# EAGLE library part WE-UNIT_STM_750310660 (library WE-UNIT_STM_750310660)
Off-Line Transformer WE-Unit STM - Nominal input voltage: 85-265 VAC - Operating temperature: -40°C to +125 °C - Isolation voltage 4 kVAC -- Especially designed for several ICs from STMicroelectronics VIPer 17H -- Universal input -- Offline-switch mode power supplies
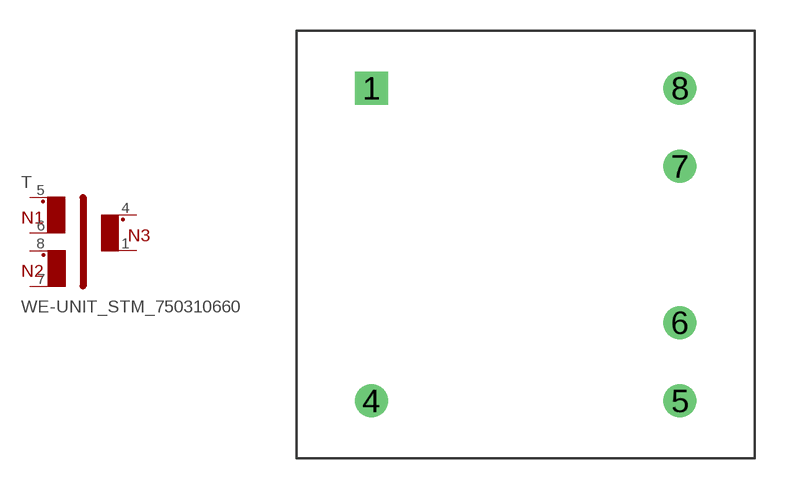
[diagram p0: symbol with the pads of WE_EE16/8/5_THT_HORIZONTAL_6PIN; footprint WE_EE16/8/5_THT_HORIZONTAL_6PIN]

Designator prefix T

## WE-UNIT_STM_750310660 (MPN: 750310660; OC_FARNELL: 1849043; OC_NEWARK: 13T9827; PACKAGE: EE16/8/5; SUPPLIER: Würth Elektronik eiSos GmbH)  [WE_EE16/8/5_THT_HORIZONTAL_6PIN]
1  5  pas
4  6  pas
5  1  pas
6  2  pas
7  4  pas
8  3  pas

## Footprint WE_EE16/8/5_THT_HORIZONTAL_6PIN (pad centres in mm)
Transformer, EE16/8/5 THT Horizontal 6 Pin
drill 1.07 square: 1 -7.525,7.62
drill 1.07: 4 -7.525,-7.62; 5 7.525,-7.62; 6 7.525,-3.81; 7 7.525,3.81; 8 7.525,7.62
